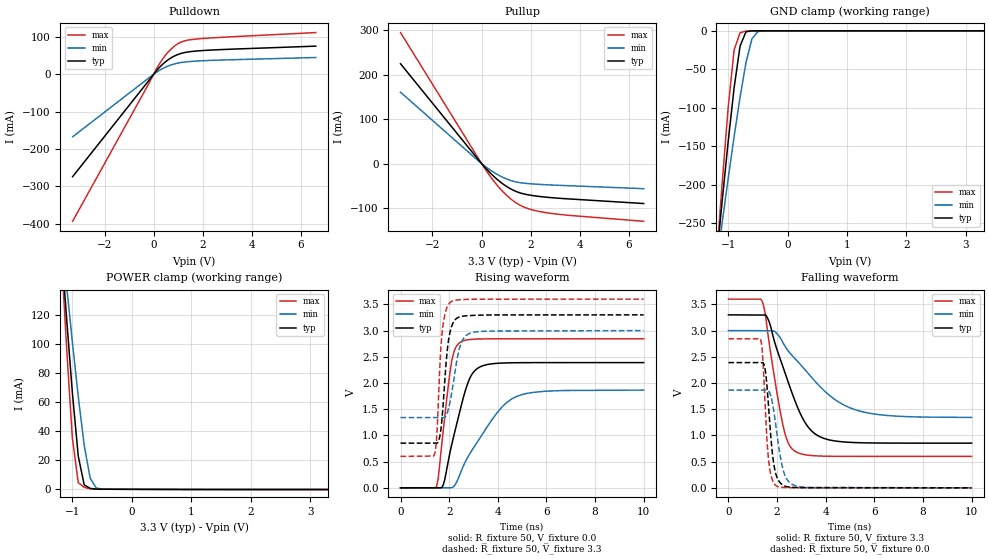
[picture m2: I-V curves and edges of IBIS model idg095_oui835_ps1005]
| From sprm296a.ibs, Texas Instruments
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[Model]   idg095_oui835_ps1005
Model_type   I/O
Vinh = 2.00
Vinl = 0.80
Enable   Active-Low
Polarity   Non-Inverting
| signals   A, GZ, Y
Vmeas = 1.5
|   typ   min   max
C_comp   5.766p   5.693p   5.808p
|   typ   min   max
[Temperature Range]   25   -40   125
|   typ   min   max
[Voltage Range]   3.30V   3.00V   3.60V
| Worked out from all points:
|   slope of the pulldown table from 0 to 0.495 V, typ, clamps not added: 14.6 ohm
|   slope of the pullup table from 0 to 0.495 V, typ, clamps not added: 17.1 ohm
|   GND clamp passes 1 mA (typ) near -0.68 V on its own axis
|   POWER clamp passes 1 mA (typ) near -0.72 V on its own axis
|   rising waveform, R_fixture 50, V_fixture 0.0: 20-80 % time 754ps typ, 1.54ns min, 419ps max; typ from 0.001 V to 2.39 V
|   falling waveform, R_fixture 50, V_fixture 3.3: 20-80 % time 1.15ns typ, 2.04ns min, 635ps max; typ from 3.3 V to 0.854 V
|   rising waveform, R_fixture 50, V_fixture 3.3: 20-80 % time 262ps typ, 376ps min, 205ps max; typ from 0.854 V to 3.3 V
|   falling waveform, R_fixture 50, V_fixture 0.0: 20-80 % time 267ps typ, 377ps min, 206ps max; typ from 2.39 V to 0.001 V
[Pulldown]
|   Voltage   I(typ)   I(min)   I(max)
-3.3V     -273.9mA   -167.3mA   -393.2mA
-200mV    -17mA      -10.01mA   -25.19mA
200mV     15.78mA    9.018mA    24.02mA
500mV     34.27mA    19.55mA    52.44mA
700mV     43.5mA     24.72mA    66.87mA
900mV     50.47mA    28.56mA    77.95mA
1.2V      57.14mA    32.16mA    88.1mA
1.8V      62.45mA    35.48mA    94.53mA
6.6V      75.19mA    44.76mA    111.5mA
[GND_clamp]
|   Voltage   I(typ)   I(min)   I(max)
-3.3V     -2.104A    -1.603A    -2.704A
-1.2V     -299.6mA   -306.5mA   -301.5mA
-1.1V     -220.2mA   -248.5mA   -196.8mA
-1V       -143.9mA   -191.9mA   -99.65mA
-900mV    -73.93mA   -137.3mA   -24.73mA
-800mV    -19.86mA   -85.99mA   -2.582mA
-700mV    -1.246mA   -41.12mA   -247.7uA
-600mV    -50.35uA   -10.34mA   -13.99uA
-500mV    -2.403uA   -939.8uA   -484.2nA
-300mV    -4.469nA   -3.168uA   -582.9pA
3.3V      222pA      897.8nA    399.7pA
[Pullup]
|   Voltage   I(typ)   I(min)   I(max)
-3.3V     224.7mA    160.6mA    295mA
100mV     -6.373mA   -4.422mA   -8.632mA
400mV     -23.87mA   -16.43mA   -32.51mA
700mV     -38.83mA   -26.47mA   -53.25mA
1.2V      -57.64mA   -38.47mA   -80.36mA
1.5V      -65mA      -42.63mA   -91.89mA
1.8V      -69.49mA   -44.77mA   -99.81mA
2.5V      -75.13mA   -47.46mA   -109.6mA
3.5V      -79.61mA   -49.93mA   -116.5mA
6.6V      -90.17mA   -56.73mA   -130.2mA
[POWER_clamp]
|   Voltage   I(typ)   I(min)   I(max)
-3.3V     1.461A     1.112A     1.882A
-1.2V     175.6mA    182.9mA    173.1mA
-1.1V     119.4mA    141.6mA    99.76mA
-1V       66.64mA    101.5mA    35.53mA
-900mV    22.67mA    63.6mA     4.516mA
-800mV    3.002mA    30.22mA    1.326mA
-700mV    612.4uA    7.671mA    368.4uA
-600mV    159.2uA    996.1uA    126.6uA
-500mV    72.14uA    150.9uA    89.15uA
3.3V      -134.4uA   -86.16uA   -207.6uA
[Ramp]
|   I(typ)   I(min)   I(max)
dV/dt_r   1.433/0.752n   1.119/1.533n   1.705/0.417n
dV/dt_f   1.468/1.154n   0.994/2.041n   1.799/0.635n
[Rising Waveform]
R_fixture = 50
V_fixture = 0.0
|  pu_on
|  TIME   V(typ)   V(min)   V(max)
0s        1.265mV    1.19mV     1.383mV
1.486ns   2.119mV    2.32mV     32.39mV
1.762ns   62.41mV    2.32mV     1.116V
2.093ns   800.8mV    2.32mV     2.385V
2.48ns    1.536V     303.1mV    2.784V
2.811ns   2.051V     622.2mV    2.828V
3.142ns   2.271V     863mV      2.838V
4.135ns   2.38V      1.522V     2.843V
4.797ns   2.387V     1.748V     2.844V
10ns      2.39V      1.865V     2.844V
[Falling Waveform]
R_fixture = 50
V_fixture = 3.3
V_fixture_min = 3.0
V_fixture_max = 3.6
|  pd_on
|  TIME   V(typ)   V(min)   V(max)
0s        3.3V       3V         3.6V
1.399ns   3.297V     2.997V     3.548V
1.68ns    3.162V     2.997V     2.747V
2.243ns   2.308V     2.77V      1.194V
2.453ns   2.024V     2.615V     862.8mV
2.735ns   1.663V     2.467V     699.7mV
3.156ns   1.244V     2.249V     632.3mV
3.578ns   1.026V     2.026V     612.2mV
5.194ns   865.1mV    1.494V     601.5mV
10ns      853.9mV    1.343V     601.3mV
[Rising Waveform]
R_fixture = 50
V_fixture = 3.3
V_fixture_min = 3.0
V_fixture_max = 3.6
|  pd_off
|  TIME   V(typ)   V(min)   V(max)
0s        853.9mV    1.342V     601.3mV
1.413ns   853.9mV    1.342V     659.6mV
1.494ns   853.9mV    1.342V     1.021V
1.629ns   1.015V     1.342V     2.428V
1.71ns    1.342V     1.342V     2.967V
1.927ns   2.643V     1.442V     3.457V
2.09ns    3.062V     1.768V     3.553V
2.442ns   3.263V     2.692V     3.589V
2.875ns   3.287V     2.952V     3.597V
10ns      3.3V       3V         3.6V
[Falling Waveform]
R_fixture = 50
V_fixture = 0.0
|  pu_off
|  TIME   V(typ)   V(min)   V(max)
0s        2.39V      1.866V     2.844V
1.313ns   2.39V      1.865V     2.844V
1.396ns   2.39V      1.865V     2.58V
1.501ns   2.284V     1.865V     1.677V
1.647ns   1.574V     1.849V     552.2mV
1.814ns   633mV      1.606V     145mV
1.981ns   220.4mV    1.08V      35.7mV
2.294ns   40.57mV    274.7mV    8.589mV
2.775ns   7.758mV    39.11mV    3.535mV
10ns      1.266mV    1.198mV    1.384mV
